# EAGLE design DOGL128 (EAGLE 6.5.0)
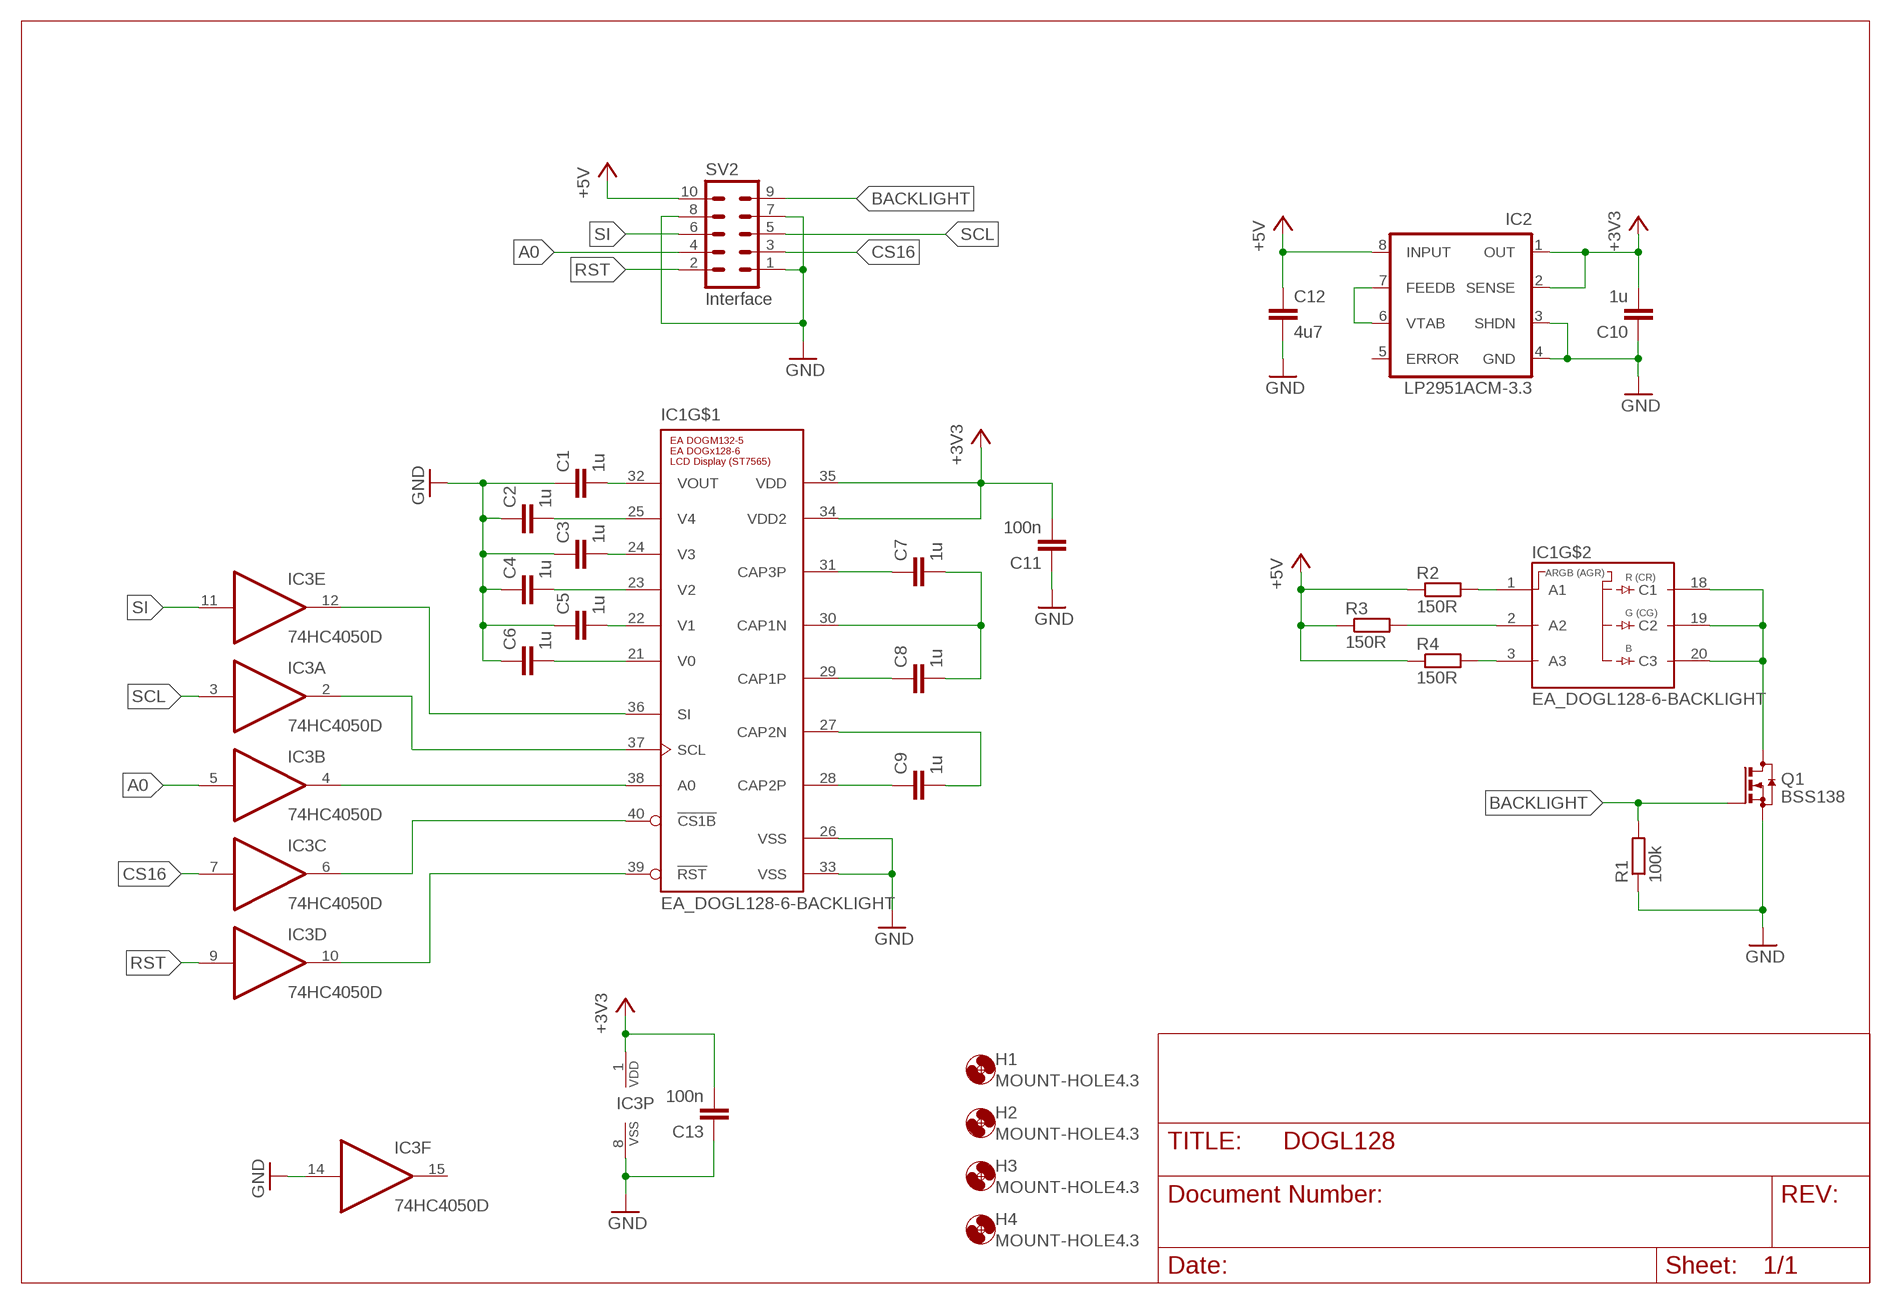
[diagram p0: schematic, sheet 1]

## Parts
C1  1u  C-EUC0805  [C0805]
C2  1u  C-EUC0805  [C0805]
C3  1u  C-EUC0805  [C0805]
C4  1u  C-EUC0805  [C0805]
C5  1u  C-EUC0805  [C0805]
C6  1u  C-EUC0805  [C0805]
C7  1u  C-EUC0805  [C0805]
C8  1u  C-EUC0805  [C0805]
C9  1u  C-EUC0805  [C0805]
C10  1u  C-EUC0805  [C0805]
C11  100n  C-EUC0805  [C0805]
C12  4u7  C-EUC0805  [C0805]
C13  100n  C-EUC0805  [C0805]
H1  MOUNT-HOLE4.3  [4,3]
H2  MOUNT-HOLE4.3  [4,3]
H3  MOUNT-HOLE4.3  [4,3]
H4  MOUNT-HOLE4.3  [4,3]
IC1  EA_DOGL128-6-BACKLIGHT  [EA_DOGL128_BACKLIGHT]
IC2  LP2951ACM-3.3  [SO-08]
IC3  74HC4050D  4050D  [SO16]
Q1  BSS138  BSS123  [SOT23]
R1  100k  R-EU_R0805  [R0805]
R2  150R  R-EU_R1206  [R1206]
R3  150R  R-EU_R1206  [R1206]
R4  150R  R-EU_R1206  [R1206]
SV2  Interface  ML10  [ML10]

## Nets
+3V3: C10.2 C11.2 C13.2 IC1.34(VDD2) IC1.35(VDD) IC2.1(OUT) IC2.2(SENSE) IC3.1(P:VDD)
+5V: C12.1 IC2.8(INPUT) R2.1 R3.1 R4.1 SV2.10
A0: IC3.5(B:I) SV2.4
BACKLIGHT: Q1.1(G) R1.2 SV2.9
CS16: IC3.7(C:I) SV2.3
GND: C1.1 C2.1 C3.1 C4.1 C5.1 C6.1 C10.1 C11.1 C12.2 C13.1 IC1.26(VSS) IC1.33(VSS) IC2.3(SHDN) IC2.4(GND) IC3.8(P:VSS) IC3.14(F:I) Q1.2(S) R1.1 SV2.1 SV2.7 SV2.8
N$1: IC1.1(A1) R2.2
N$2: IC1.2(A2) R3.2
N$3: IC1.3(A3) R4.2
N$4: IC1.18(C1) IC1.19(C2) IC1.20(C3) Q1.3(D)
N$5: IC2.6(VTAB) IC2.7(FEEDB)
N$10: IC1.36(SI) IC3.12(E:O)
N$11: IC1.37(SCL) IC3.2(A:O)
N$12: IC1.38(A0) IC3.4(B:O)
N$16: IC1.40(!CS1B) IC3.6(C:O)
N$17: IC1.39(!RST) IC3.10(D:O)
N$18: C3.2 IC1.24(V3)
N$19: C1.2 IC1.32(VOUT)
N$20: C2.2 IC1.25(V4)
N$21: C4.2 IC1.23(V2)
N$22: C5.2 IC1.22(V1)
N$23: C6.2 IC1.21(V0)
N$24: C7.1 IC1.31(CAP3P)
N$25: C8.1 IC1.29(CAP1P)
N$26: C9.1 IC1.28(CAP2P)
N$27: C7.2 C8.2 IC1.30(CAP1N)
N$28: C9.2 IC1.27(CAP2N)
RST: IC3.9(D:I) SV2.2
SCL: IC3.3(A:I) SV2.5
SI: IC3.11(E:I) SV2.6
Unconnected: IC2.5(ERROR) IC3.15(F:O)

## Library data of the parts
C1-C13 = resistor:C-EU: CAPACITOR, European symbol
H1-H4 = holes:MOUNT-HOLE: MOUNTING HOLE with drill center marker
IC1 = EA-DOG-LCD:EA_DOGL128-6: EA DOGL128-6 mit LED-Beleuchtung EA LED68X51-xxx Grafikdisplay COG 128x64 Pixel inkl.Kontroller (ST 7565R) Hersteller: ELECTRONIC ASSEMBLY GmbH http://www.lcd-module.de
IC2 = v-reg:LP2951?*: Series of Adjustable Micropower Voltage Regulators Source: http://cache.national.com/ds/LP/LP2950.pdf
IC3 = 40xx:4050: Hex non-inverting BUFFER
Q1 = transistor-small-signal:BSS123: N-CHANNEL MOS FET
R1-R4 = rcl:R-EU_: RESISTOR, European symbol
SV2 = con-harting-ml:ML10: HARTING; OC_FARNELL: unknown; OC_NEWARK: unknown

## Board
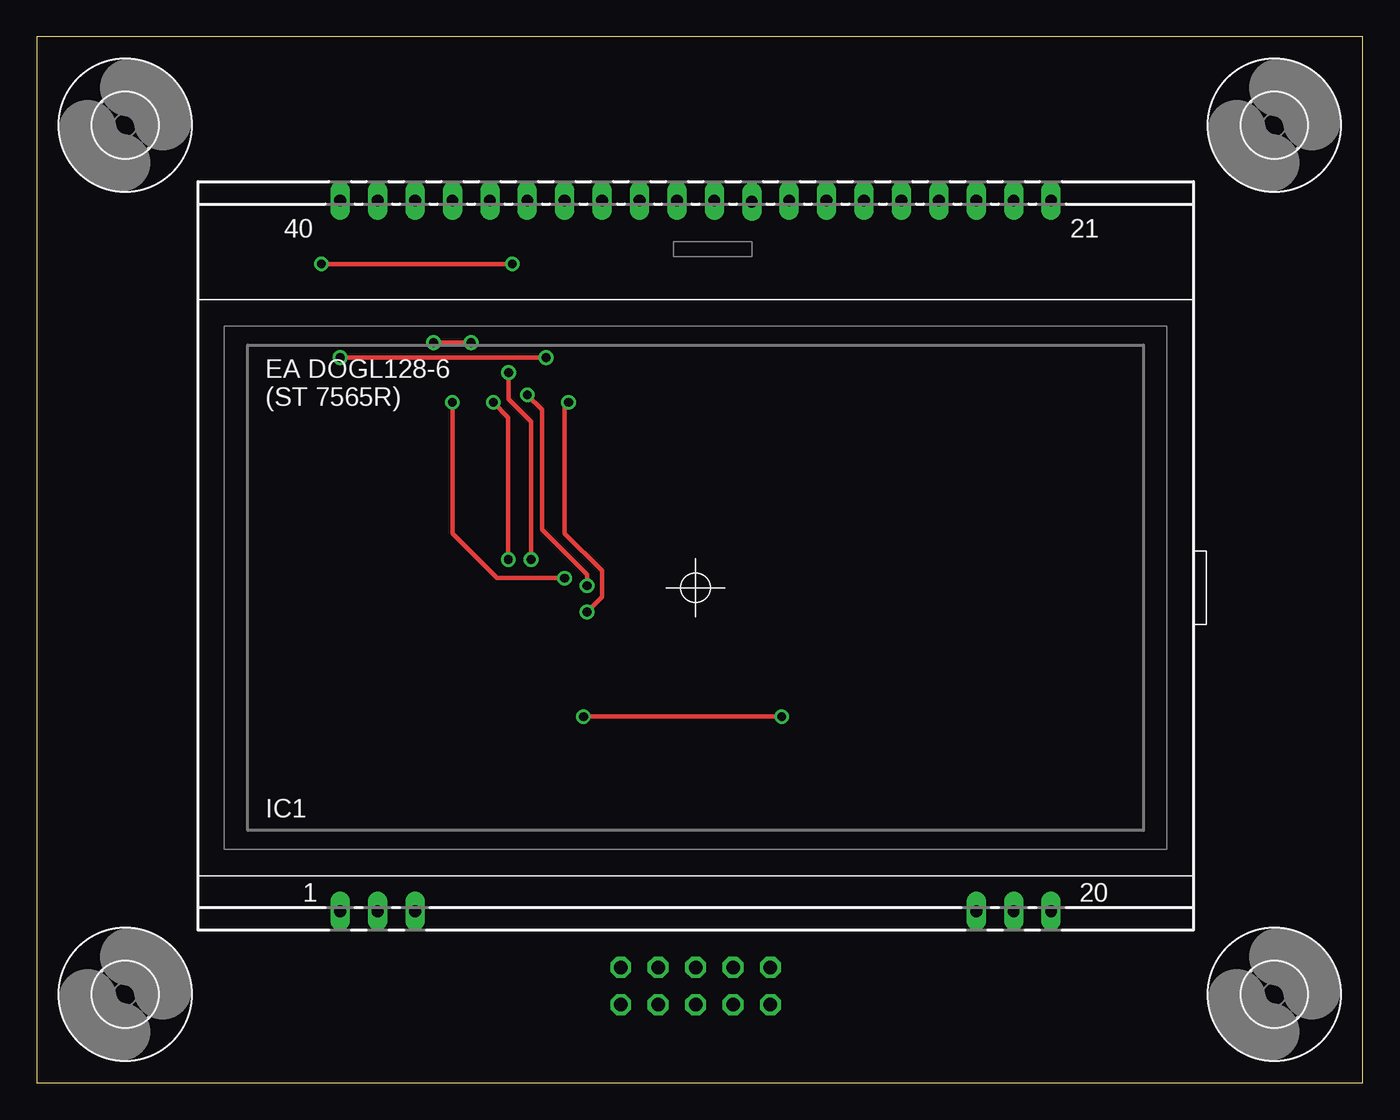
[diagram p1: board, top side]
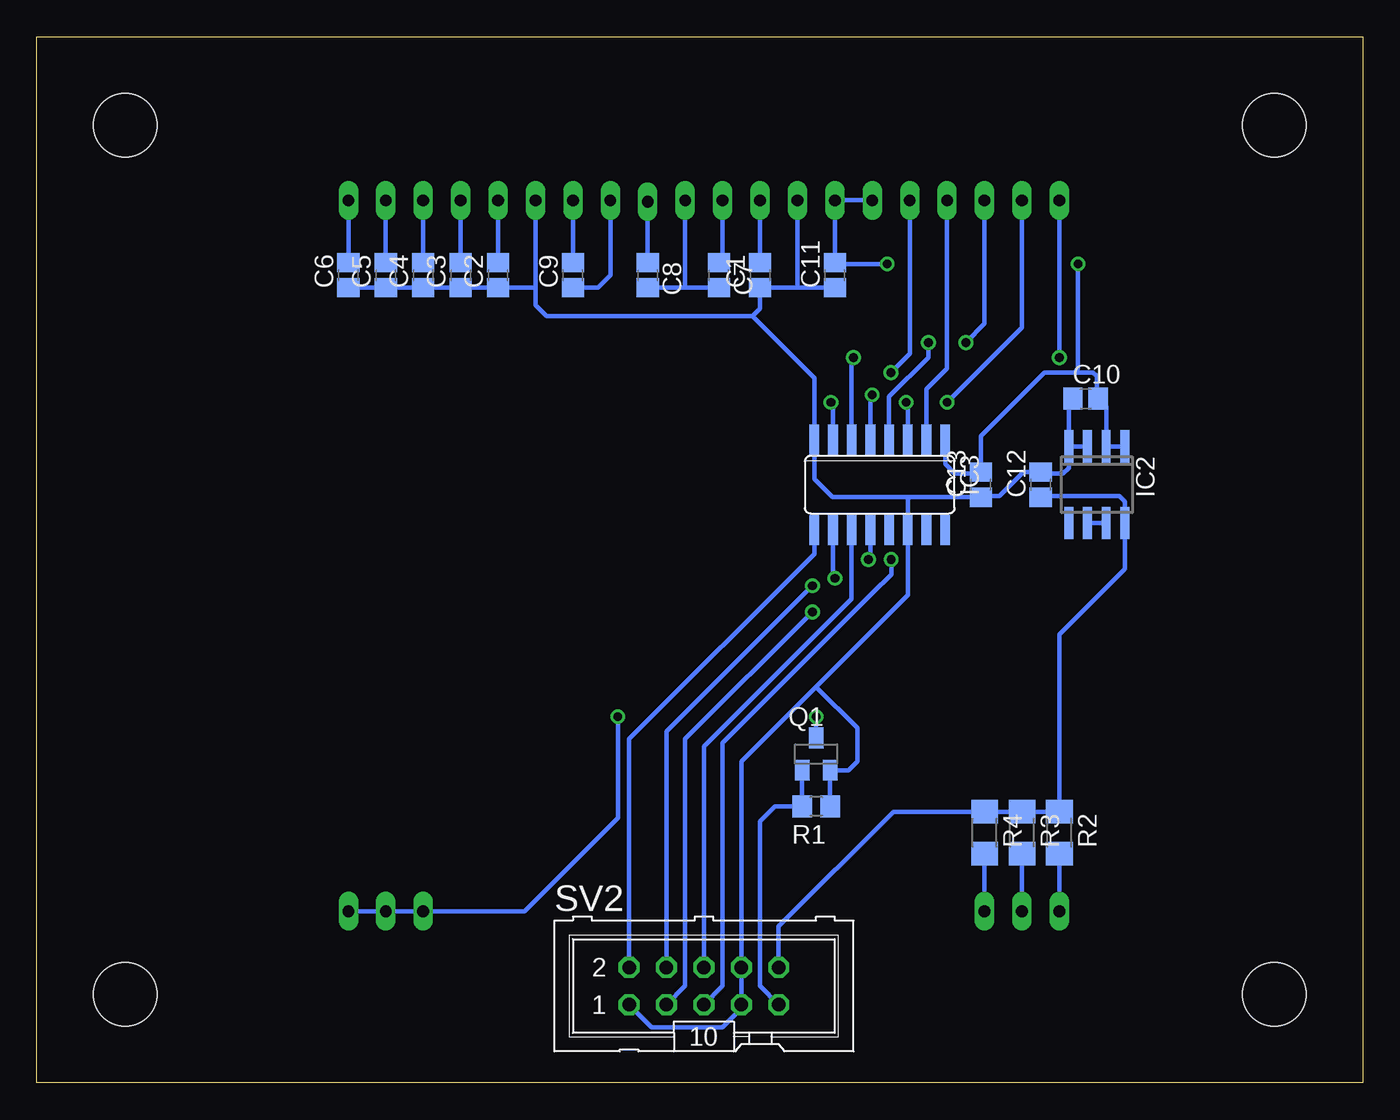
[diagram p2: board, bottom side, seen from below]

Size 90 x 71 mm. Coordinates in mm from the lower left corner, seen from the top.
Outline: 0,0 90,0 90,71 0,71 0,0
Copper layers (1*16): Top 0.035mm / dielectric 1.5mm / Bottom 0.035mm
Design rules "default *": minimum track width 0.3mm, minimum drill 0.6mm, track to track 0.3mm, track to pad 0.3mm, pad to pad 0.3mm, via to via 0.3mm, smd to smd 8mil, copper to edge 40mil, drill to drill 8mil, minimum pad ring 10mil, minimum via ring 8mil, stop-mask expansion 4mil, vias tented up to drill 0mil, thermal gap 10mil

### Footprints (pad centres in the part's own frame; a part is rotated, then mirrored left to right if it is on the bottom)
C0805 = smd 1.3 x 1.5: 1 -0.85,0; 2 0.85,0
4,3 = hole 4.3: 0,0
EA_DOGL128_BACKLIGHT = drill 0.8 long: 1 0,0; 2 2.54,0; 3 5.08,0; 18 43.18,0; 19 45.72,0; 20 48.26,0; 21 48.26,48.26; 22 45.72,48.26; 23 43.18,48.26; 24 40.64,48.26; 25 38.1,48.26; 26 35.56,48.26; 27 33.02,48.26; 28 30.48,48.26; 29 27.94,48.17; 30 25.4,48.26; 31 22.86,48.26; 32 20.32,48.26; 33 17.78,48.26; 34 15.24,48.26; 35 12.7,48.26; 36 10.16,48.26; 37 7.62,48.26; 38 5.08,48.26; 39 2.54,48.26; 40 0,48.26
SO-08 = smd 0.6 x 2.2: 1 -1.905,-2.6; 2 -0.635,-2.6; 3 0.635,-2.6; 4 1.905,-2.6; 5 1.905,2.6; 6 0.635,2.6; 7 -0.635,2.6; 8 -1.905,2.6
SO16 = smd 0.66 x 2.032: 1 -4.445,-3.073; 2 -3.175,-3.073; 3 -1.905,-3.073; 4 -0.635,-3.073; 5 0.635,-3.073; 6 1.905,-3.073; 7 3.175,-3.073; 8 4.445,-3.073; 9 4.445,3.073; 10 3.175,3.073; 11 1.905,3.073; 12 0.635,3.073; 13 -0.635,3.073; 14 -1.905,3.073; 15 -3.175,3.073; 16 -4.445,3.073
SOT23 = smd 1 x 1.4: 1 -0.95,-1.1; 2 0.95,-1.1; 3 0,1.1
R0805 = smd 1.3 x 1.5: 1 -0.95,0; 2 0.95,0
R1206 = smd 1.6 x 1.803: 1 -1.422,0; 2 1.422,0
ML10 = drill 0.914 octagon: 1 -5.08,-1.27; 2 -5.08,1.27; 3 -2.54,-1.27; 4 -2.54,1.27; 5 0,-1.27; 6 0,1.27; 7 2.54,-1.27; 8 2.54,1.27; 9 5.08,-1.27; 10 5.08,1.27

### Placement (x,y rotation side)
C1  40.91,54.82 90 bottom
C2  58.69,54.82 90 bottom
C3  61.23,54.82 90 bottom
C4  63.77,54.82 90 bottom
C5  66.31,54.82 90 bottom
C6  68.85,54.82 90 bottom
C7  43.7,54.82 270 bottom
C8  48.53,54.82 270 bottom
C9  53.61,54.82 90 bottom
C10  18.81,46.44 0 bottom
C11  35.83,54.82 90 bottom
C12  21.86,40.6 90 bottom
C13  25.92,40.6 90 bottom
H1  84,6 0 top
H2  6,6 0 top
H3  84,65 0 top
H4  6,65 0 top
IC1  20.59,11.64 0 top
IC2  18.05,40.6 180 bottom
IC3  32.78,40.6 180 bottom
Q1  37.1,22.31 0 bottom
R1  37.1,18.75 180 bottom
R2  20.59,16.97 270 bottom
R3  23.13,16.97 270 bottom
R4  25.67,16.97 270 bottom
SV2  44.72,6.56 0 bottom

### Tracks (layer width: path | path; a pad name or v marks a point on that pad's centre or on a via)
+3V3  (via drill 0.6)
  Top 0.305: v32.27,55.58 v19.32,55.58
  Bottom 0.305: IC1.35 IC1.34 C11.2 35.74,55.58 v32.27,55.58 | IC2.1 IC2.2 17.41,45.89 C10.2 18.05,46.53 18.05,47.96 18.3,48.22 19.57,48.22 | IC3.1 28.34,41.99 27.7,41.36 26.01,41.36 C13.2 25.92,43.9 21.61,48.22 19.57,48.22 | v19.32,55.58 19.32,48.47 19.57,48.22
+5V
  Bottom 0.305: SV2.10 39.64,10.62 31.87,18.4 R4.1 R3.1 R2.1 20.59,30.44 16.14,34.88 IC2.8 16.14,39.45 16.53,39.83 21.77,39.83 C12.1
A0  (via drill 0.6)
  Top 0.305: v37.35,33.74 37.35,34.48 34.29,37.55 34.29,45.69 v33.29,46.69
  Bottom 0.305: SV2.4 47.26,23.83 v37.35,33.74 | IC3.5 33.42,46.56 v33.29,46.69
BACKLIGHT
  Bottom 0.305: Q1.1 R1.2 39.89,18.75 40.91,17.74 40.91,6.56 SV2.9
CS16  (via drill 0.6)
  Top 0.305: v37.35,31.96 38.35,32.96 38.35,34.75 35.81,37.29 35.81,45.91 v36.08,46.18
  Bottom 0.305: SV2.3 45.99,6.56 45.99,23.32 v37.35,31.96 | IC3.7 35.96,46.06 v36.08,46.18
GND
  Bottom 0.305: C6.1 C5.1 C4.1 C3.1 C2.1 56.24,53.97 56.15,54.06 | C11.1 38.37,53.97 | 38.37,53.97 C1.1 40.91,52.53 41.42,52.03 | 41.42,52.03 55.39,52.03 56.15,52.79 56.15,54.06 | IC1.33 38.37,53.97 | 36.15,18.82 Q1.2 34.9,21.21 34.31,21.8 34.31,24.09 37.1,26.88 | R1.1 36.15,18.82 | 36.15,18.82 35.83,18.5 | IC2.3 IC2.4 | IC2.4 19.95,41.74 20.34,41.36 21.77,41.36 C12.2 23.04,41.45 24.65,39.83 25.84,39.83 C13.1 30.75,39.75 | IC2.4 19.95,46.14 C10.1 | 30.75,39.75 36,39.75 37.23,40.98 IC3.8 37.23,47.83 41.42,52.03 | 30.75,39.75 30.88,39.62 IC3.14 30.88,33.1 37.1,26.88 | IC1.26 56.15,54.06 | SV2.1 48.28,3.77 43.45,3.77 42.18,5.04 SV2.7 SV2.8 42.18,21.8 37.1,26.88
N$1
  Bottom 0.305: IC1.1 R2.2
N$2
  Bottom 0.305: R3.2 IC1.2
N$3
  Bottom 0.305: R4.2 IC1.3
N$4  (via drill 0.6)
  Top 0.305: v37.1,24.85 v50.56,24.85
  Bottom 0.305: IC1.20 IC1.19 IC1.18 56.9,11.64 50.55,17.99 50.55,24.83 v50.56,24.85 | Q1.3 v37.1,24.85
N$5
  Bottom 0.305: IC2.7 IC2.6
N$10  (via drill 0.6)
  Top 0.305: v33.54,35.52 33.54,44.9 32.02,46.42 v32.02,48.22
  Bottom 0.305: IC1.36 30.75,49.49 v32.02,48.22 | IC3.12 33.42,35.64 v33.54,35.52
N$11
  Bottom 0.305: IC3.2 29.61,47.07 28.21,48.47 IC1.37
N$12  (via drill 0.6)
  Top 0.305: v26.94,50.25 v29.48,50.25
  Bottom 0.305: IC1.38 25.67,51.52 v26.94,50.25 | v29.48,50.25 29.48,49.23 32.15,46.56 IC3.4
N$16  (via drill 0.6)
  Top 0.305: v20.59,49.23 v34.56,49.23
  Bottom 0.305: IC1.40 v20.59,49.23 | IC3.6 34.69,49.11 v34.56,49.23
N$17  (via drill 0.6)
  Top 0.305: v28.21,46.18 28.21,37.28 31.24,34.25 v35.83,34.25
  Bottom 0.305: IC1.39 23.13,51.26 v28.21,46.18 | IC3.10 35.96,34.37 v35.83,34.25
N$18
  Bottom 0.305: IC1.24 C3.2
N$19
  Bottom 0.305: IC1.32 C1.2
N$20
  Bottom 0.305: IC1.25 C2.2
N$21
  Bottom 0.305: IC1.23 C4.2
N$22
  Bottom 0.305: IC1.22 C5.2
N$23
  Bottom 0.305: IC1.21 C6.2
N$24
  Bottom 0.305: IC1.31 43.45,55.92 C7.1
N$25
  Bottom 0.305: C8.1 IC1.29
N$26
  Bottom 0.305: C9.1 51.92,53.97 51.07,54.82 IC1.28
N$27
  Bottom 0.305: C8.2 45.99,53.97 | 45.99,53.97 C7.2 | IC1.30 45.99,53.97
N$28
  Bottom 0.305: IC1.27 C9.2
RST
  Bottom 0.305: SV2.2 49.8,23.32 37.23,35.9 IC3.9
SCL  (via drill 0.6)
  Top 0.305: v32,35.52 32,45.17 v30.99,46.18
  Bottom 0.305: SV2.5 43.45,6.56 43.45,23.07 33.29,33.23 33.27,33.23 32,34.5 v32,35.52 | IC3.3 30.88,46.07 v30.99,46.18
SI
  Bottom 0.305: SV2.6 44.72,22.82 34.69,32.85 IC3.11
